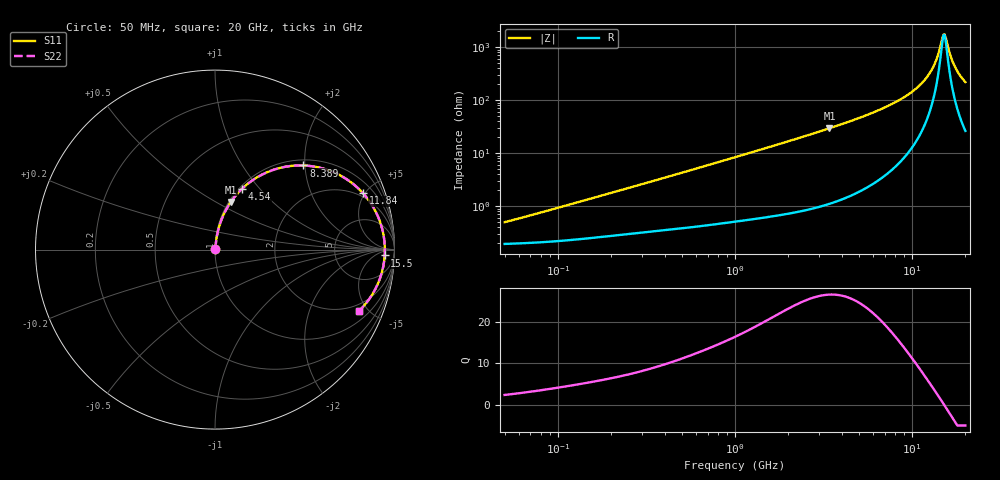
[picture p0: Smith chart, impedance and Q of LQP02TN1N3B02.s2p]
!Murata Part Number: LQP02TN1N3B02
!These Parameters are Measured in Series Mode Connection
!  o--[Z]--o
!Port1  Port2
!  o-------o
!Freq. Start=50[MHz] Stop=20[GHz], 401[Steps]
# Hz S RI R 50
!Freq.(Hz) S11(Real) S11(Imag) S21(Real) S21(Imag) S12(Real) S12(Imag) S22(Real) S22(Imag)
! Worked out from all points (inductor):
!   401 points, 50 MHz to 20 GHz, reference 50 ohm
!   read as one part in series: L = 1.45 nH near 66.46 MHz
!   highest Q = 26.6 at 3.415 GHz (marker M1), where L = 1.37 nH
!   self-resonance near 15.16 GHz
!   S11 on the Smith chart (normalised r, x): 50 MHz: 1.00, +0.01; 4.54 GHz: 1.03, +0.81; 8.389 GHz: 1.13, +1.96; 11.84 GHz: 1.71, +4.84; 15.5 GHz: 26, -16; 20 GHz: 1.52, -4.34
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5e7  0.00195 0.00456  0.998 -0.00456  0.998 -0.00456  0.00195 0.00456
1.364002e8  0.00254 0.0121  0.9975 -0.0121  0.9975 -0.0121  0.00254 0.0121
3.721004e8  0.0044 0.0316  0.9956 -0.0316  0.9956 -0.0316  0.0044 0.0316
1e9  0.0119 0.082  0.9881 -0.082  0.9881 -0.082  0.0119 0.082
2.728004e9  0.058 0.2152  0.942 -0.2152  0.942 -0.2152  0.058 0.2152
3.415248e9  0.0878 0.2649  0.9122 -0.2649  0.9122 -0.2649  0.0878 0.2649
4.539627e9  0.1514 0.3395  0.8486 -0.3395  0.8486 -0.3395  0.1514 0.3395
5.856089e9  0.2487 0.4107  0.7513 -0.4107  0.7513 -0.4107  0.2487 0.4107
7.442007e9  0.3947 0.462  0.6053 -0.462  0.6053 -0.462  0.3947 0.462
8.389408e9  0.4922 0.4687  0.5078 -0.4687  0.5078 -0.4687  0.4922 0.4687
1.019291e10  0.6796 0.4224  0.3204 -0.4224  0.3204 -0.4224  0.6796 0.4224
1.183995e10  0.824 0.3147  0.176 -0.3147  0.176 -0.3147  0.824 0.3147
1.257102e10  0.8723 0.2515  0.1277 -0.2515  0.1277 -0.2515  0.8723 0.2515
1.334722e10  0.9106 0.1781  0.0894 -0.1781  0.0894 -0.1781  0.9106 0.1781
1.396067e10  0.9309 0.1178  0.0691 -0.1178  0.0691 -0.1178  0.9309 0.1178
1.482269e10  0.9451 0.0327  0.0549 -0.0327  0.0549 -0.0327  0.9451 0.0327
1.527346e10  0.9464 -0.0107  0.0536 0.0107  0.0536 0.0107  0.9464 -0.0107
1.550395e10  0.9455 -0.0324  0.0545 0.0324  0.0545 0.0324  0.9455 -0.0324
1.646126e10  0.9321 -0.1177  0.0679 0.1177  0.0679 0.1177  0.9321 -0.1177
1.721783e10  0.9123 -0.1785  0.0877 0.1785  0.0877 0.1785  0.9123 -0.1785
1.855685e10  0.8635 -0.2696  0.1365 0.2696  0.1365 0.2696  0.8635 -0.2696
2e10  0.7997 -0.3443  0.2003 0.3443  0.2003 0.3443  0.7997 -0.3443
